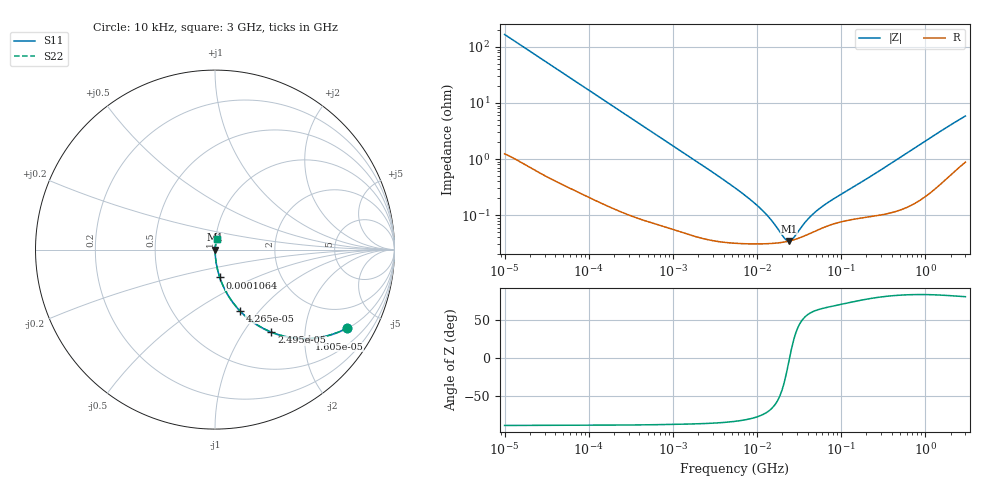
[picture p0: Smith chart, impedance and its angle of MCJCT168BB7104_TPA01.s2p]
! MCJCT168BB7104_TPA01  S-PARAMETER MODEL  ( Standard Model )
! Model Generated by TAIYO YUDEN Corporation (http://www.ty-top.com)
! Version 1.0
! TAIYO YUDEN Control No. 220601
! Copyright(c) 2015 TAIYO YUDEN CO.,LTD. All Rights Reserved.
! Product Description (link to TY-COMPAS)
! https://ds.yuden.co.jp/TYCOMPAS/or/detail?pn=MCJCT168BB7104KTPA01&u=M
! Products Name : Multilayer Ceramic Capacitors
! Characteristics :
!  Capacitance : 0.1 [uF] , Rated Voltage : 25 [V] , TCC : X7R
!  Case Size : 1.6 x 0.8 / 0.063 x 0.031 [mm/inch] , Thickness : 0.8 / 0.031 [mm/inch]
!  (Conditions: Temperature = 25 [degC] , DC Bias Voltage = 0 [V])
! External Node Assignments :
!  1  o---| |---o  2
! GND o---------o GND
! Frequency Range : 10kHz  -  3GHz  [ 401 STEP ]
# MHZ S RI R 50
! Freq[MHz].  S11 Real  S11 Imag  S21 Real  S21 Imag  S12 Real  S12 Imag  S22 Real  S22 Imag
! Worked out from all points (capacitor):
!   401 points, 10 kHz to 3 GHz, reference 50 ohm
!   read as one part in series: C = 94.8 nF near 10.65 kHz
!   lowest |Z| = 34.4 mohm at 24.11 MHz (marker M1)
!   series resonance near 24.39 MHz, so ESL is about 450 pH
!   S11 on the Smith chart (normalised r, x): 10 kHz: 1.02, -3.35; 16.05 kHz: 1.02, -2.09; 24.95 kHz: 1.01, -1.35; 42.65 kHz: 1.01, -0.79; 106.4 kHz: 1.00, -0.32; 3 GHz: 1.02, +0.12
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0.01  0.7359 -0.4372  0.2641 0.4372  0.2641 0.4372  0.7359 -0.4372
0.016047  0.5229 -0.4954  0.4771 0.4954  0.4771 0.4954  0.5229 -0.4954
0.024951  0.3146 -0.46  0.6854 0.46  0.6854 0.46  0.3146 -0.46
0.033138  0.2079 -0.4013  0.7921 0.4013  0.7921 0.4013  0.2079 -0.4013
0.042645  0.138 -0.3401  0.862 0.3401  0.862 0.3401  0.138 -0.3401
0.082683  0.0425 -0.1959  0.9575 0.1959  0.9575 0.1959  0.0425 -0.1959
0.106405  0.0267 -0.1551  0.9733 0.1551  0.9733 0.1551  0.0267 -0.1551
0.241531  0.0061 -0.0702  0.9939 0.0702  0.9939 0.0702  0.0061 -0.0702
0.683653  0.0013 -0.0251  0.9987 0.0251  0.9987 0.0251  0.0013 -0.0251
5.477226  0.000323 -0.00304  0.9997 0.00304  0.9997 0.00304  0.000323 -0.00304
8.252149  0.00031 -0.00189  0.9997 0.00189  0.9997 0.00189  0.00031 -0.00189
11.31085  0.000308 -0.00122  0.9997 0.00122  0.9997 0.00122  0.000308 -0.00122
15.02209  0.000312 -0.000727  0.9997 0.000727  0.9997 0.000727  0.000312 -0.000727
21.24962  0.000331 -0.000198  0.9997 0.000198  0.9997 0.000198  0.000331 -0.000198
24.10585  0.000344 -1.63e-05  0.9997 1.63e-05  0.9997 1.63e-05  0.000344 -1.63e-05
27.34599  0.000362 0.000163  0.9996 -0.000163  0.9996 -0.000163  0.000362 0.000163
36.31858  0.000422 0.000567  0.9996 -0.000567  0.9996 -0.000567  0.000422 0.000567
45.28751  0.00049 0.000885  0.9995 -0.000885  0.9995 -0.000885  0.00049 0.000885
72.67256  0.000659 0.00162  0.9993 -0.00162  0.9993 -0.00162  0.000659 0.00162
374.4521  0.00114 0.00793  0.9989 -0.00793  0.9989 -0.00793  0.00114 0.00793
1547.292  0.00462 0.0315  0.9954 -0.0315  0.9954 -0.0315  0.00462 0.0315
3000  0.012 0.0568  0.988 -0.0568  0.988 -0.0568  0.012 0.0568
